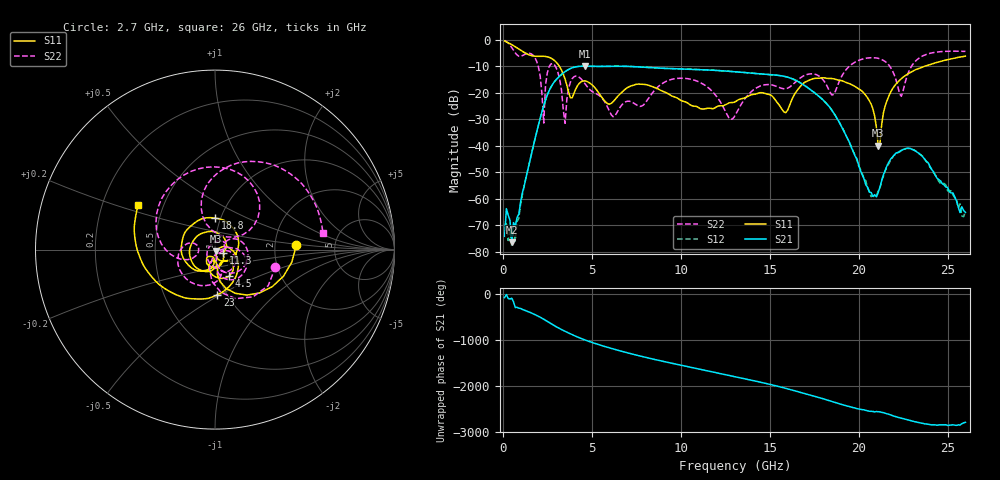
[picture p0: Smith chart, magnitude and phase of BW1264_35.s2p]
!Keysight Technologies,N5245B,MY57181159,A.13.60.06
!Date: Friday, December 18, 2020 23:53:48
!Correction: S11(Full 2 Port(1,2))
!S21(Full 2 Port(1,2))
!S12(Full 2 Port(1,2))
!S22(Full 2 Port(1,2))
!S2P File: Measurements: S11, S21, S12, S22:
# Hz S  dB  R 50
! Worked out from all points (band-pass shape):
!   260 points, 100 MHz to 26 GHz, reference 50 ohm
!   highest |S21| = -9.93 dB at 4.6 GHz (marker M1); lowest = -76.4 dB at 500 MHz (marker M2)
!   |S21| within 3 dB of the highest: 3.32 GHz to 14.66 GHz (11.34 GHz wide, 126 % of centre)
!   lowest |S11| = -39.9 dB at 21.1 GHz (marker M3), VSWR 1.02, Z = 50.4 - j0.914 ohm
!   |S11| at or under -10 dB: 3.181 GHz to 23.69 GHz (20.51 GHz wide, 153 % of centre)
!   |S22| runs from -31.5 to -0.2 dB; largest |S21 - S12| = 0.00057
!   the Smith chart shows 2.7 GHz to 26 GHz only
!   S11 on the Smith chart (normalised r, x): 2.7 GHz: 2.65, +0.16; 4.5 GHz: 1.12, -0.34; 11.3 GHz: 1.10, -0.04; 18.8 GHz: 0.94, +0.34; 23 GHz: 0.90, -0.49; 26 GHz: 0.36, +0.23
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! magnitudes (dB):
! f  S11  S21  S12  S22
! 100 MHz  -0.4  -74.2  -69.7  -0.2
! 200 MHz  -0.7  -63.7  -69.5  -0.6
! 500 MHz  -1.8  -76.4  -77.9  -2.9
! 1.9 GHz  -6.2  -34.8  -34.9  -8.1
! 2.3 GHz  -6.2  -24.8  -24.8  -31.4
! 2.7 GHz  -6.9  -17.9  -17.9  -9.1
! 3.5 GHz  -14.8  -12.0  -12.0  -31.5
! 3.8 GHz  -21.9  -10.8  -10.8  -15.9
! 4.5 GHz  -15.5  -9.9  -9.9  -15.5
! 4.6 GHz  -15.5  -9.9  -9.9  -16.4
! 6.2 GHz  -23.3  -9.9  -9.9  -29.0
! 8.8 GHz  -18.8  -10.7  -10.7  -17.3
! 11.3 GHz  -26.1  -11.3  -11.3  -16.9
! 13.1 GHz  -23.2  -12.0  -12.0  -28.0
! 17.4 GHz  -14.7  -19.3  -19.3  -12.8
! 18.8 GHz  -15.1  -29.8  -29.8  -17.5
! 20.5 GHz  -21.9  -55.6  -55.9  -6.8
! 21.1 GHz  -39.9  -57.6  -57.1  -7.0
! 21.7 GHz  -21.2  -46.2  -46.7  -9.5
! 22.4 GHz  -14.6  -41.8  -41.6  -21.3
! 23 GHz  -12.0  -41.3  -41.4  -9.6
! 26 GHz  -6.1  -65.2  -64.8  -4.3
